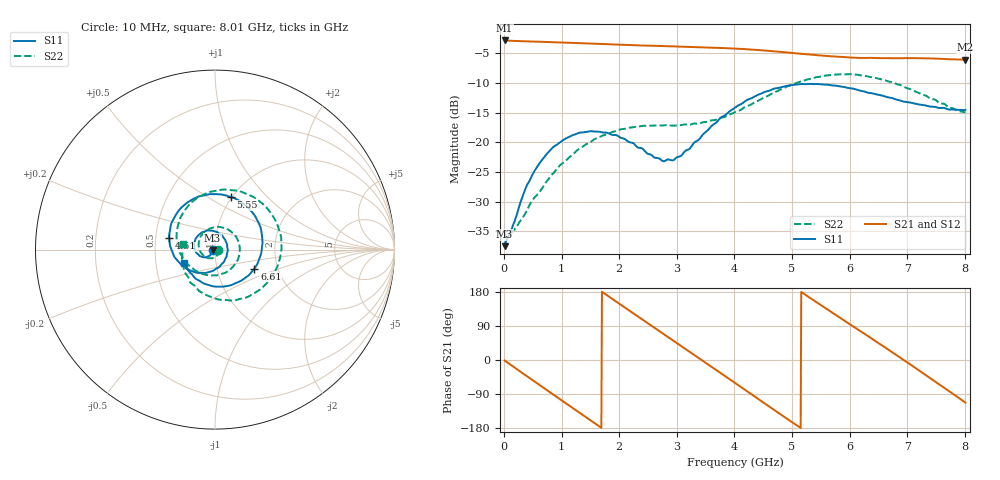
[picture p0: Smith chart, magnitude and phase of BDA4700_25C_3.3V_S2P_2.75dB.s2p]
!Agilent Technologies,E5071B,MY42404982,A.09.10
!Date: Mon Oct 20 18:04:08 2025
!Data & Calibration Information:
!Freq	S11:SOLT2(ON)	S21:SOLT2(ON)	S12:SOLT2(ON)	S22:SOLT2(ON)
# Hz S RI R 50
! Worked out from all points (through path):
!   801 points, 10 MHz to 8.01 GHz, reference 50 ohm
!   highest |S21| = -2.86 dB at 10 MHz (marker M1); lowest = -6.1 dB at 8.01 GHz (marker M2)
!   group delay of S21, straight-line fit = 288 ps
!   lowest |S11| = -37.5 dB at 10 MHz (marker M3), VSWR 1.03, Z = 48.7 - j0.167 ohm
!   |S11| at or under -10 dB: start of sweep to end of sweep
!   |S22| runs from -36.1 to -8.5 dB; largest |S21 - S12| = 0.0083
!   S11 on the Smith chart (normalised r, x): 10 MHz: 0.97, -0.00; 4.51 GHz: 0.59, +0.08; 5.55 GHz: 0.99, +0.64; 6.61 GHz: 1.52, -0.34; 8.01 GHz: 0.70, -0.11
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1e7  -0.0132 -0.00171  0.719 -0.0155  0.7187 -0.0162  0.0169 -0.00155
3.3e8  -0.0229 -0.0278  0.5761 -0.4122  0.5758 -0.4124  0.0181 -0.0148
7.1e8  -0.0633 -0.0424  0.1708 -0.6778  0.1707 -0.6781  -0.00461 -0.0444
1.02e9  -0.1018 -0.0199  -0.22 -0.6549  -0.2203 -0.655  -0.0515 -0.0424
1.35e9  -0.1166 0.0318  -0.5472 -0.4071  -0.5473 -0.4077  -0.0898 0.0124
1.92e9  -0.0477 0.1048  -0.6124 0.2606  -0.6128 0.2605  -0.00943 0.1232
2.32e9  0.0258 0.0867  -0.2811 0.5912  -0.2809 0.5911  0.1011 0.0905
2.68e9  0.0666 0.0308  0.1335 0.6329  0.1326 0.6328  0.138 -0.0149
3.06e9  0.0588 -0.0487  0.5 0.3973  0.4957 0.4013  0.0802 -0.1137
3.36e9  0.0143 -0.1021  0.6264 0.0826  0.6268 0.0827  -0.00195 -0.1431
3.67e9  -0.0652 -0.1292  0.5667 -0.2618  0.5664 -0.2635  -0.0895 -0.1258
4.01e9  -0.168 -0.1004  0.3024 -0.5353  0.3031 -0.5345  -0.1671 -0.0649
4.51e9  -0.2558 0.0626  -0.2316 -0.5448  -0.2316 -0.5461  -0.213 0.1059
4.93e9  -0.1899 0.231  -0.5232 -0.2239  -0.5226 -0.2269  -0.1214 0.2709
5.35e9  -0.0101 0.309  -0.5128 0.1857  -0.514 0.1827  0.095 0.3307
5.55e9  0.087 0.2935  -0.4093 0.3441  -0.4103 0.3429  0.2084 0.296
6.07e9  0.2545 0.1219  0.0202 0.5142  0.0196 0.5168  0.3699 0.041
6.61e9  0.2193 -0.106  0.4262 0.2832  0.4256 0.282  0.2412 -0.2293
6.68e9  0.2003 -0.1295  0.4565 0.228  0.4573 0.2271  0.2071 -0.2494
7.23e9  0.0143 -0.2066  0.4407 -0.2562  0.4408 -0.2568  -0.0518 -0.251
7.62e9  -0.1051 -0.1641  0.1622 -0.4758  0.1616 -0.4764  -0.1695 -0.1264
8.01e9  -0.1725 -0.0727  -0.1883 -0.457  -0.1867 -0.4582  -0.1757 0.0308
